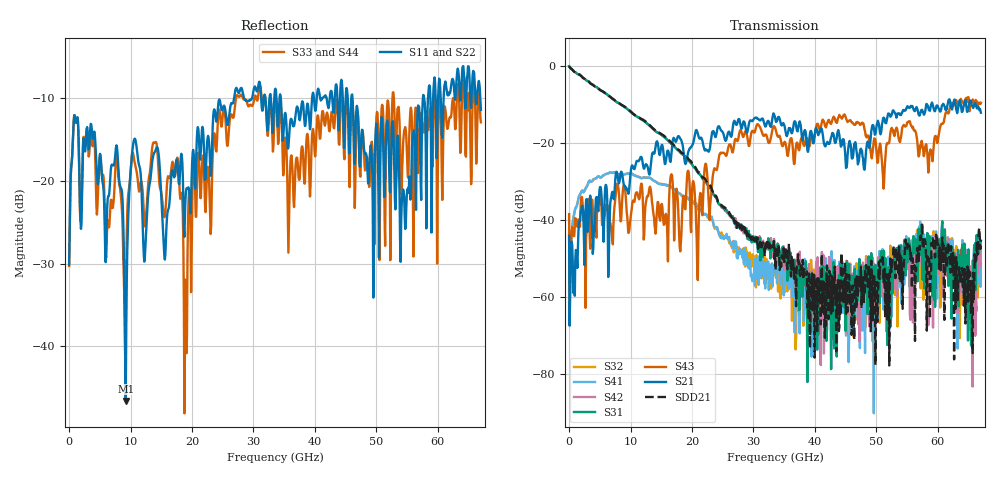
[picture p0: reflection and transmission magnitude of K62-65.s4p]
!Agilent Technologies,N5247A,US50470101,A.10.25.02
!Agilent N5247A: A.10.25.02
!Date: Tuesday, May 12, 2015 13:44:23
!Correction: Sdd11(Full 4 Port(1,2,3,4))
!Sdc11(Full 4 Port(1,2,3,4))
!Sdd12(Full 4 Port(1,2,3,4))
!Sdc12(Full 4 Port(1,2,3,4))
!Scd11(Full 4 Port(1,2,3,4))
!Scc11(Full 4 Port(1,2,3,4))
!Scd12(Full 4 Port(1,2,3,4))
!Scc12(Full 4 Port(1,2,3,4))
!Sdd21(Full 4 Port(1,2,3,4))
!Sdc21(Full 4 Port(1,2,3,4))
!Sdd22(Full 4 Port(1,2,3,4))
!Sdc22(Full 4 Port(1,2,3,4))
!Scd21(Full 4 Port(1,2,3,4))
!Scc21(Full 4 Port(1,2,3,4))
!Scd22(Full 4 Port(1,2,3,4))
!Scc22(Full 4 Port(1,2,3,4))
!Balanced Topology: BBAL
!S4P File: Measurements: <Sdd11,Sdc11,Sdd12,Sdc12>,
!<Scd11,Scc11,Scd12,Scc12>,
!<Sdd21,Sdc21,Sdd22,Sdc22>,
!<Scd21,Scc21,Scd22,Scc22>:
# Hz S  dB  R 50
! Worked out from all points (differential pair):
!   801 points, 10 MHz to 67 GHz, reference 50 ohm
!   strongest paths, dB at 10 MHz, 16.76 GHz, 33.51 GHz, 50.25 GHz, 67 GHz:
!     S21: -44.1, -20.8, -13.4, -14.2, -12.2
!     S43: -38.5, -28.5, -16.0, -25.1, -9.6
!     S31: -0.1, -20.4, -47.8, -58.5, -45.4
!     S42: -0.1, -20.4, -47.4, -55.0, -51.4
!     S41: -44.7, -31.8, -51.8, -65.9, -45.5
!     S32: -43.6, -31.7, -51.7, -58.9, -52.3
!   taken as a pair (ports 1,2 in; 3,4 out), SDD21 dB: -0.1, -20.2, -47.4, -62.5, -45.2
!   lowest |S11| = -46.6 dB at 9.221 GHz (marker M1), VSWR 1.01, Z = 49.5 - j0.0456 ohm
!   |S11| at or under -10 dB: start of sweep to 26.84 GHz; 34.45 GHz to 39.54 GHz (5.091 GHz wide, 13.8 % of centre); 46.11 GHz to 57.57 GHz (11.46 GHz wide, 22.1 % of centre)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
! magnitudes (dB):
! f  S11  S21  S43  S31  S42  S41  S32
! 10 MHz  -30.2  -44.1  -38.5  -0.1  -0.1  -44.7  -43.6
! 9.221 GHz  -46.6  -32.0  -34.0  -10.9  -10.9  -28.0  -28.1
! 10.64 GHz  -14.9  -26.8  -35.2  -12.8  -12.8  -28.5  -28.4
! 18.93 GHz  -22.3  -25.5  -37.2  -23.6  -23.7  -34.1  -34.1
! 24.55 GHz  -10.3  -16.2  -22.8  -36.0  -36.1  -44.3  -44.1
! 39.03 GHz  -12.1  -20.0  -20.7  -56.9  -51.4  -61.7  -65.4
! 67 GHz  -11.4  -12.2  -9.6  -45.4  -51.4  -45.5  -52.3
